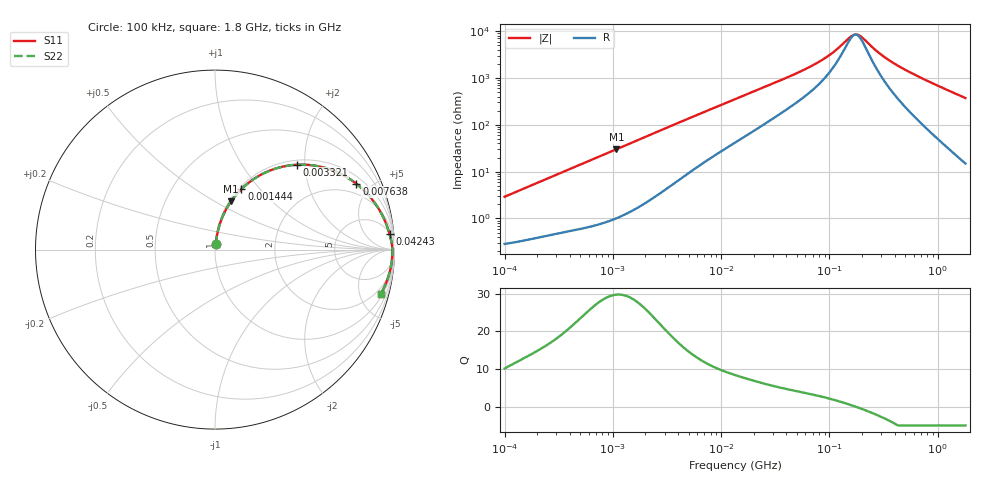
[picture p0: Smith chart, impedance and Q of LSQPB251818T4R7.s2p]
! LSQPB251818T4R7  S-PARAMETER MODEL  ( General Type )
! Model Generated by TAIYO YUDEN Corporation (http://www.ty-top.com)
! Version 2.0
! TAIYO YUDEN Control No. 100810NG19SB-FKC
! Copyright(c) 2009 TAIYO YUDEN CO.,LTD. All Rights Reserved.
! Product Description (link to TY-COMPAS)
! https://ds.yuden.co.jp/TYCOMPAS/or/detail?pn=LSQPB251818T4R7M&u=M
! Products Name : Inductors
! Characteristics :
!  Inductance : 4.7 uH , SRF(min) : 100 MHz , DC Resistance(max) : 0.299 Ohm
!  Rated Current : Saturation :1250 mA , Temp Rise : 750 mA (40 degC)
!  Case Size : 2.5 x 1.8 / 0.098 x 0.071 [mm/inch] , Thickness : 1.8 / 0.071 [mm/inch]
!  (Conditions: Temperature = 25 degC , DC Bias Current/Voltage = 0A / 0V)
! External Node Assignments :
!  1  o---GGG---o  2
! GND o---------o GND
! Frequency Range : 0.1MHz  -  1800MHz  [ 402 STEP ]
# MHz S RI R 50
! Freq[MHz].  S11 Real  S11 Imag  S21 Real  S21 Imag  S12 Real  S12 Imag  S22 Real  S22 Imag
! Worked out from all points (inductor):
!   401 points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, 100 kHz to 1.8 GHz, reference 50 ohm
!   read as one part in series: L = 4.59 uH near 105 kHz
!   highest Q = 29.7 at 1.076 MHz (marker M1), where L = 4.43 uH
!   self-resonance near 173.8 MHz
!   S11 on the Smith chart (normalised r, x): 100 kHz: 1.01, +0.06; 1.444 MHz: 1.03, +0.80; 3.321 MHz: 1.09, +1.83; 7.638 MHz: 1.36, +4.09; 42.43 MHz: 6, +21; 1.8 GHz: 1.30, -7.46
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0.1  0.00369 0.0288  0.9963 -0.0288  0.9963 -0.0288  0.00369 0.0288
0.247521  0.00915 0.0695  0.9909 -0.0695  0.9909 -0.0695  0.00915 0.0695
0.516129  0.0262 0.14  0.9738 -0.14  0.9738 -0.14  0.0262 0.14
1.076226  0.09 0.2698  0.91 -0.2698  0.91 -0.2698  0.09 0.2698
1.443982  0.1471 0.3374  0.8529 -0.3374  0.8529 -0.3374  0.1471 0.3374
1.937403  0.2325 0.4038  0.7675 -0.4038  0.7675 -0.4038  0.2325 0.4038
2.66389  0.3577 0.4573  0.6423 -0.4573  0.6423 -0.4573  0.3577 0.4573
3.320932  0.4579 0.4729  0.5421 -0.4729  0.5421 -0.4729  0.4579 0.4729
4.795486  0.624 0.4523  0.376 -0.4523  0.376 -0.4523  0.624 0.4523
7.637621  0.7878 0.3667  0.2122 -0.3667  0.2122 -0.3667  0.7878 0.3667
13.41641  0.8998 0.2465  0.1002 -0.2465  0.1002 -0.2465  0.8998 0.2465
23.56755  0.9501 0.1522  0.0499 -0.1522  0.0499 -0.1522  0.9501 0.1522
42.42587  0.9724 0.087  0.0276 -0.087  0.0276 -0.087  0.9724 0.087
69.24595  0.9815 0.0503  0.0185 -0.0503  0.0185 -0.0503  0.9815 0.0503
97.57284  0.9853 0.0299  0.0147 -0.0299  0.0147 -0.0299  0.9853 0.0299
155.4012  0.988 0.00563  0.012 -0.00563  0.012 -0.00563  0.988 0.00563
175.6488  0.9884 -0.000523  0.0116 0.000523  0.0116 0.000523  0.9884 -0.000523
198.5346  0.9886 -0.00673  0.0114 0.00673  0.0114 0.00673  0.9886 -0.00673
272.9811  0.9885 -0.0237  0.0115 0.0237  0.0115 0.0237  0.9885 -0.0237
357.3983  0.9877 -0.0399  0.0123 0.0399  0.0123 0.0399  0.9877 -0.0399
692.4421  0.9804 -0.0944  0.0196 0.0944  0.0196 0.0944  0.9804 -0.0944
1800  0.9245 -0.2449  0.0755 0.2449  0.0755 0.2449  0.9245 -0.2449
